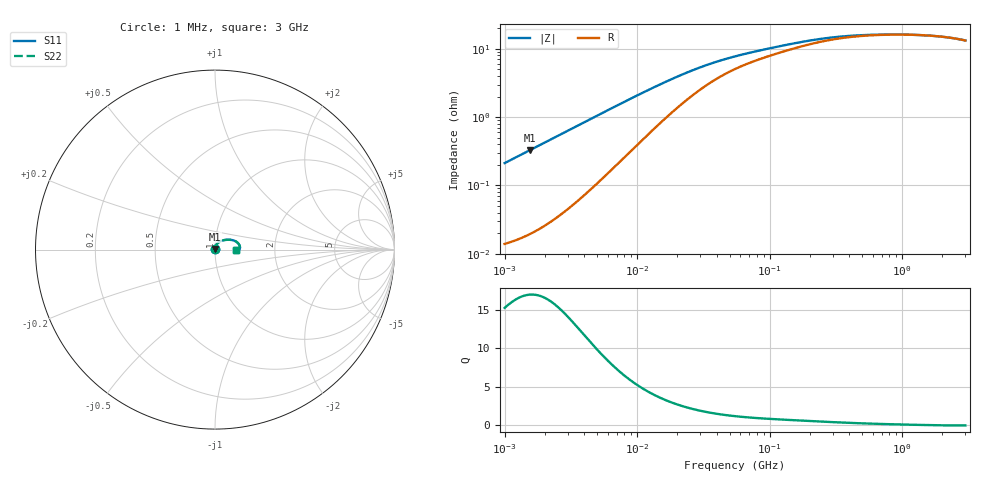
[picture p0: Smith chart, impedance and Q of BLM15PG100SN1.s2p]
! BLM15PG100SN1
# Hz S RI R 50
!Freq.(Hz) S11(Real) S11(Imag) S21(Real) S21(Imag) S12(Real) S12(Imag) S22(Real) S22(Imag)
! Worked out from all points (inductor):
!   401 points, 1 MHz to 3 GHz, reference 50 ohm
!   read as one part in series: L = 33.6 nH near 1.041 MHz
!   highest Q = 16.9 at 1.553 MHz (marker M1), where L = 33.6 nH
!   self-resonance near 1.621 GHz
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1000000  0.000143 0.00211  0.9999 -0.00211  0.9999 -0.00211  0.000143 0.00211
1040844  0.000147 0.0022  0.9999 -0.0022  0.9999 -0.0022  0.000147 0.0022
1553251  0.000204 0.00328  0.9998 -0.00328  0.9998 -0.00328  0.000204 0.00328
3823119  0.000731 0.00803  0.9993 -0.00803  0.9993 -0.00803  0.000731 0.00803
8513927  0.00318 0.0174  0.9968 -0.0174  0.9968 -0.0174  0.00318 0.0174
1.461624e7  0.00861 0.0281  0.9914 -0.0281  0.9914 -0.0281  0.00861 0.0281
2.095589e7  0.0158 0.0367  0.9842 -0.0367  0.9842 -0.0367  0.0158 0.0367
2.886629e7  0.0255 0.0441  0.9745 -0.0441  0.9745 -0.0441  0.0255 0.0441
3.976269e7  0.0377 0.0498  0.9623 -0.0498  0.9623 -0.0498  0.0377 0.0498
5.477226e7  0.0511 0.0531  0.9489 -0.0531  0.9489 -0.0531  0.0511 0.0531
7.395247e7  0.0638 0.0545  0.9362 -0.0545  0.9362 -0.0545  0.0638 0.0545
1.081723e8  0.08 0.0548  0.92 -0.0548  0.92 -0.0548  0.08 0.0548
1.550909e8  0.0959 0.0531  0.9041 -0.0531  0.9041 -0.0531  0.0959 0.0531
2.094008e8  0.1091 0.0491  0.8909 -0.0491  0.8909 -0.0491  0.1091 0.0491
2.827291e8  0.1207 0.0426  0.8793 -0.0426  0.8793 -0.0426  0.1207 0.0426
3.894533e8  0.13 0.0338  0.87 -0.0338  0.87 -0.0338  0.13 0.0338
5.473095e8  0.1362 0.0242  0.8638 -0.0242  0.8638 -0.0242  0.1362 0.0242
8.005644e8  0.1391 0.0143  0.8609 -0.0143  0.8609 -0.0143  0.1391 0.0143
1.194682e9  0.1385 0.0055  0.8615 -0.0055  0.8615 -0.0055  0.1385 0.0055
1.712864e9  0.1342 -0.000851  0.8658 0.000851  0.8658 0.000851  0.1342 -0.000851
2.266846e9  0.1276 -0.00406  0.8724 0.00406  0.8724 0.00406  0.1276 -0.00406
3e9  0.117 -0.00418  0.883 0.00418  0.883 0.00418  0.117 -0.00418
